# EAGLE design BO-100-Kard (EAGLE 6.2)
PLPB#: PLPB-0046; REV: X1
Assembly variants: build

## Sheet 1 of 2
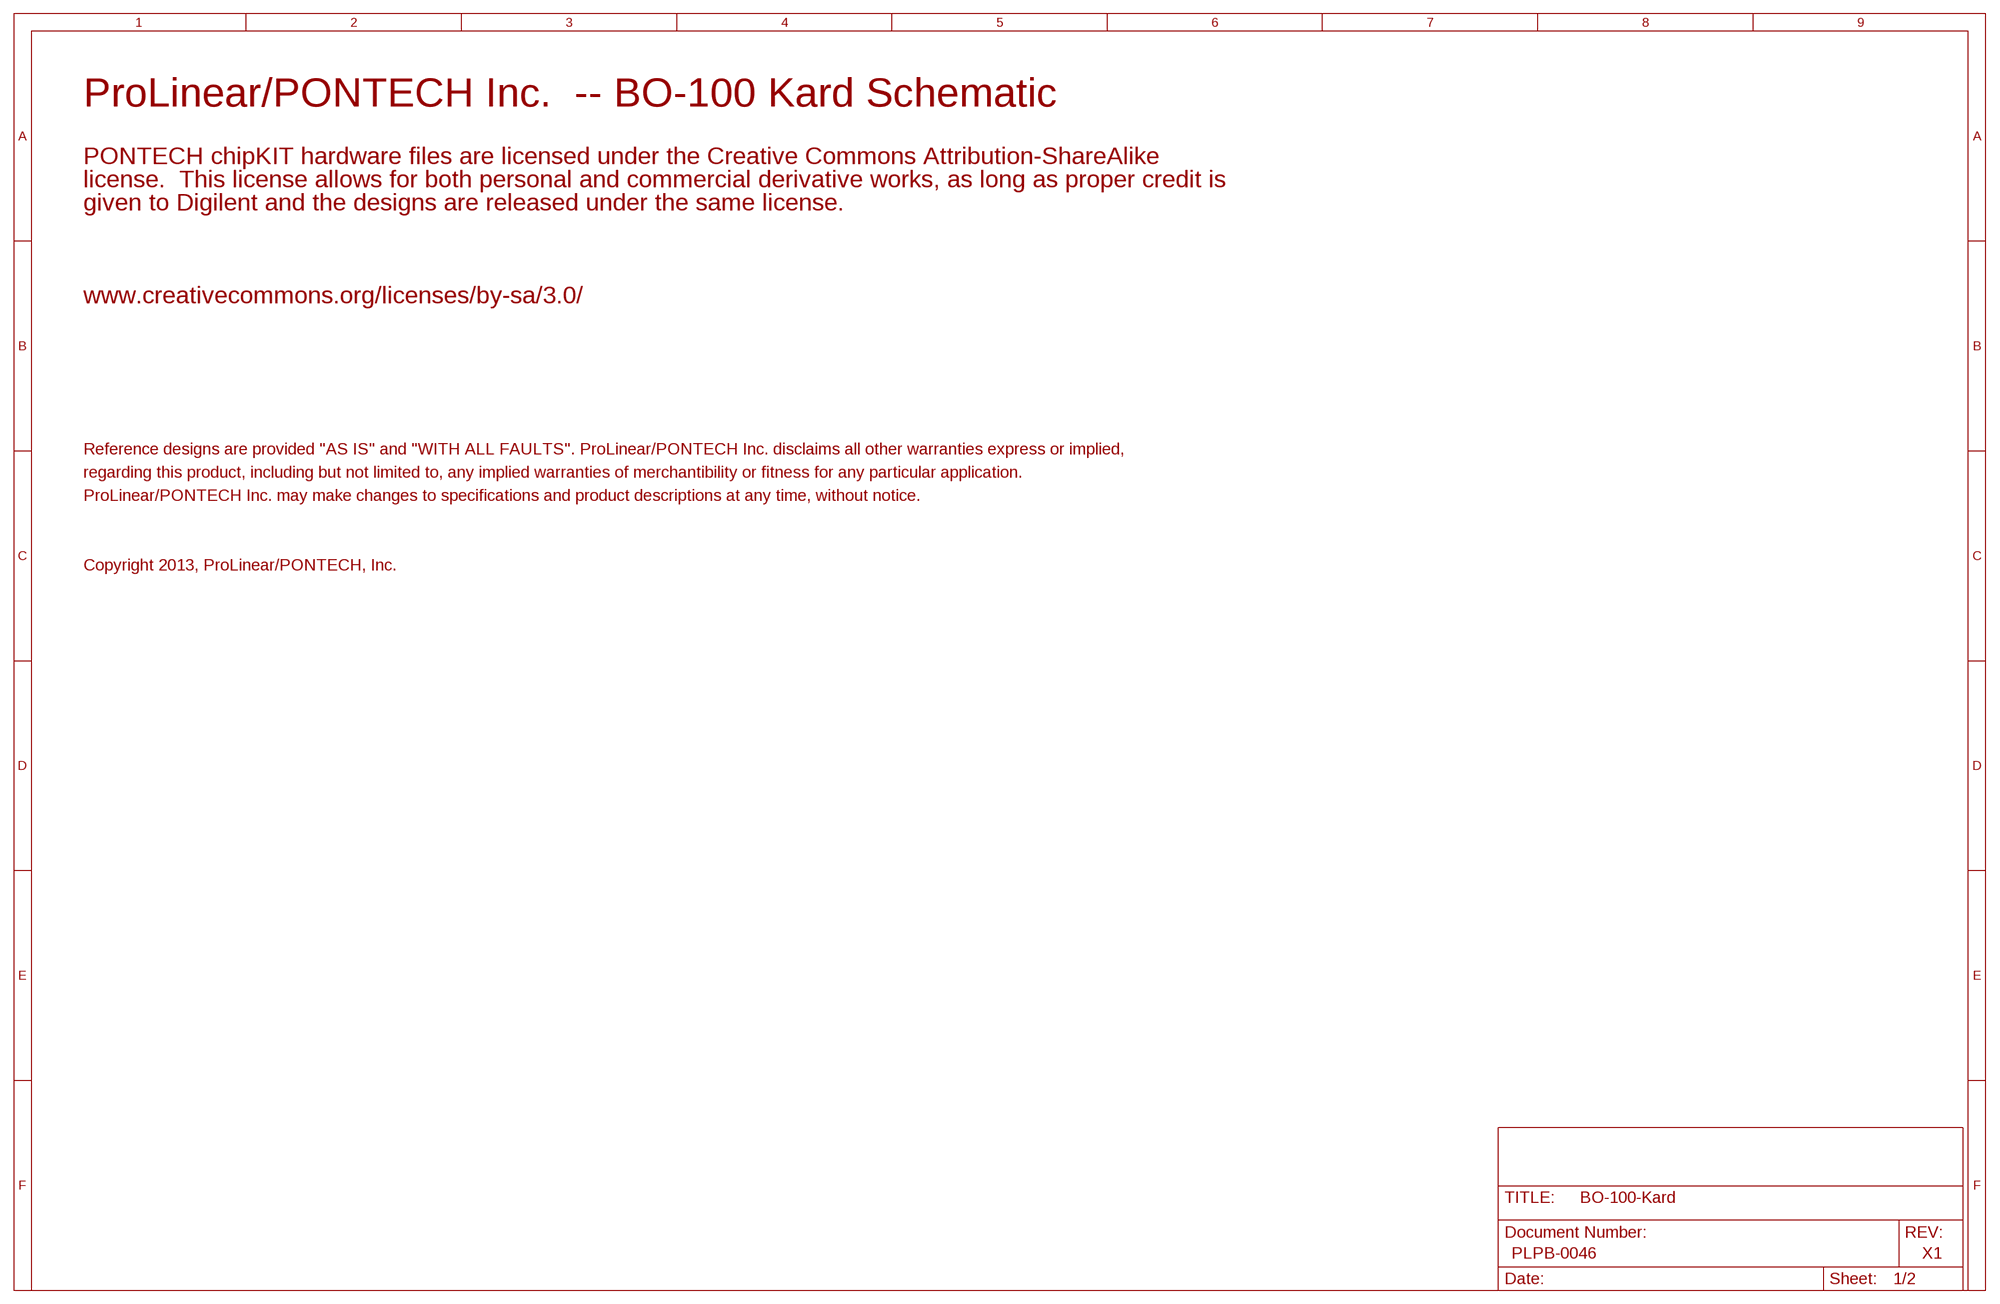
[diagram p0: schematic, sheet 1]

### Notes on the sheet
- ProLinear/PONTECH Inc.  -- BO-100 Kard Schematic
- PONTECH chipKIT hardware files are licensed under the Creative Commons Attribution-ShareAlike
- license.  This license allows for both personal and commercial derivative works, as long as proper credit is
- given to Digilent and the designs are released under the same license.
- www.creativecommons.org/licenses/by-sa/3.0/
- Reference designs are provided "AS IS" and "WITH ALL FAULTS". ProLinear/PONTECH Inc. disclaims all other warranties express or implied,
- regarding this product, including but not limited to, any implied warranties of merchantibility or fitness for any particular application.
- ProLinear/PONTECH Inc. may make changes to specifications and product descriptions at any time, without notice.
- Copyright 2013, ProLinear/PONTECH, Inc.

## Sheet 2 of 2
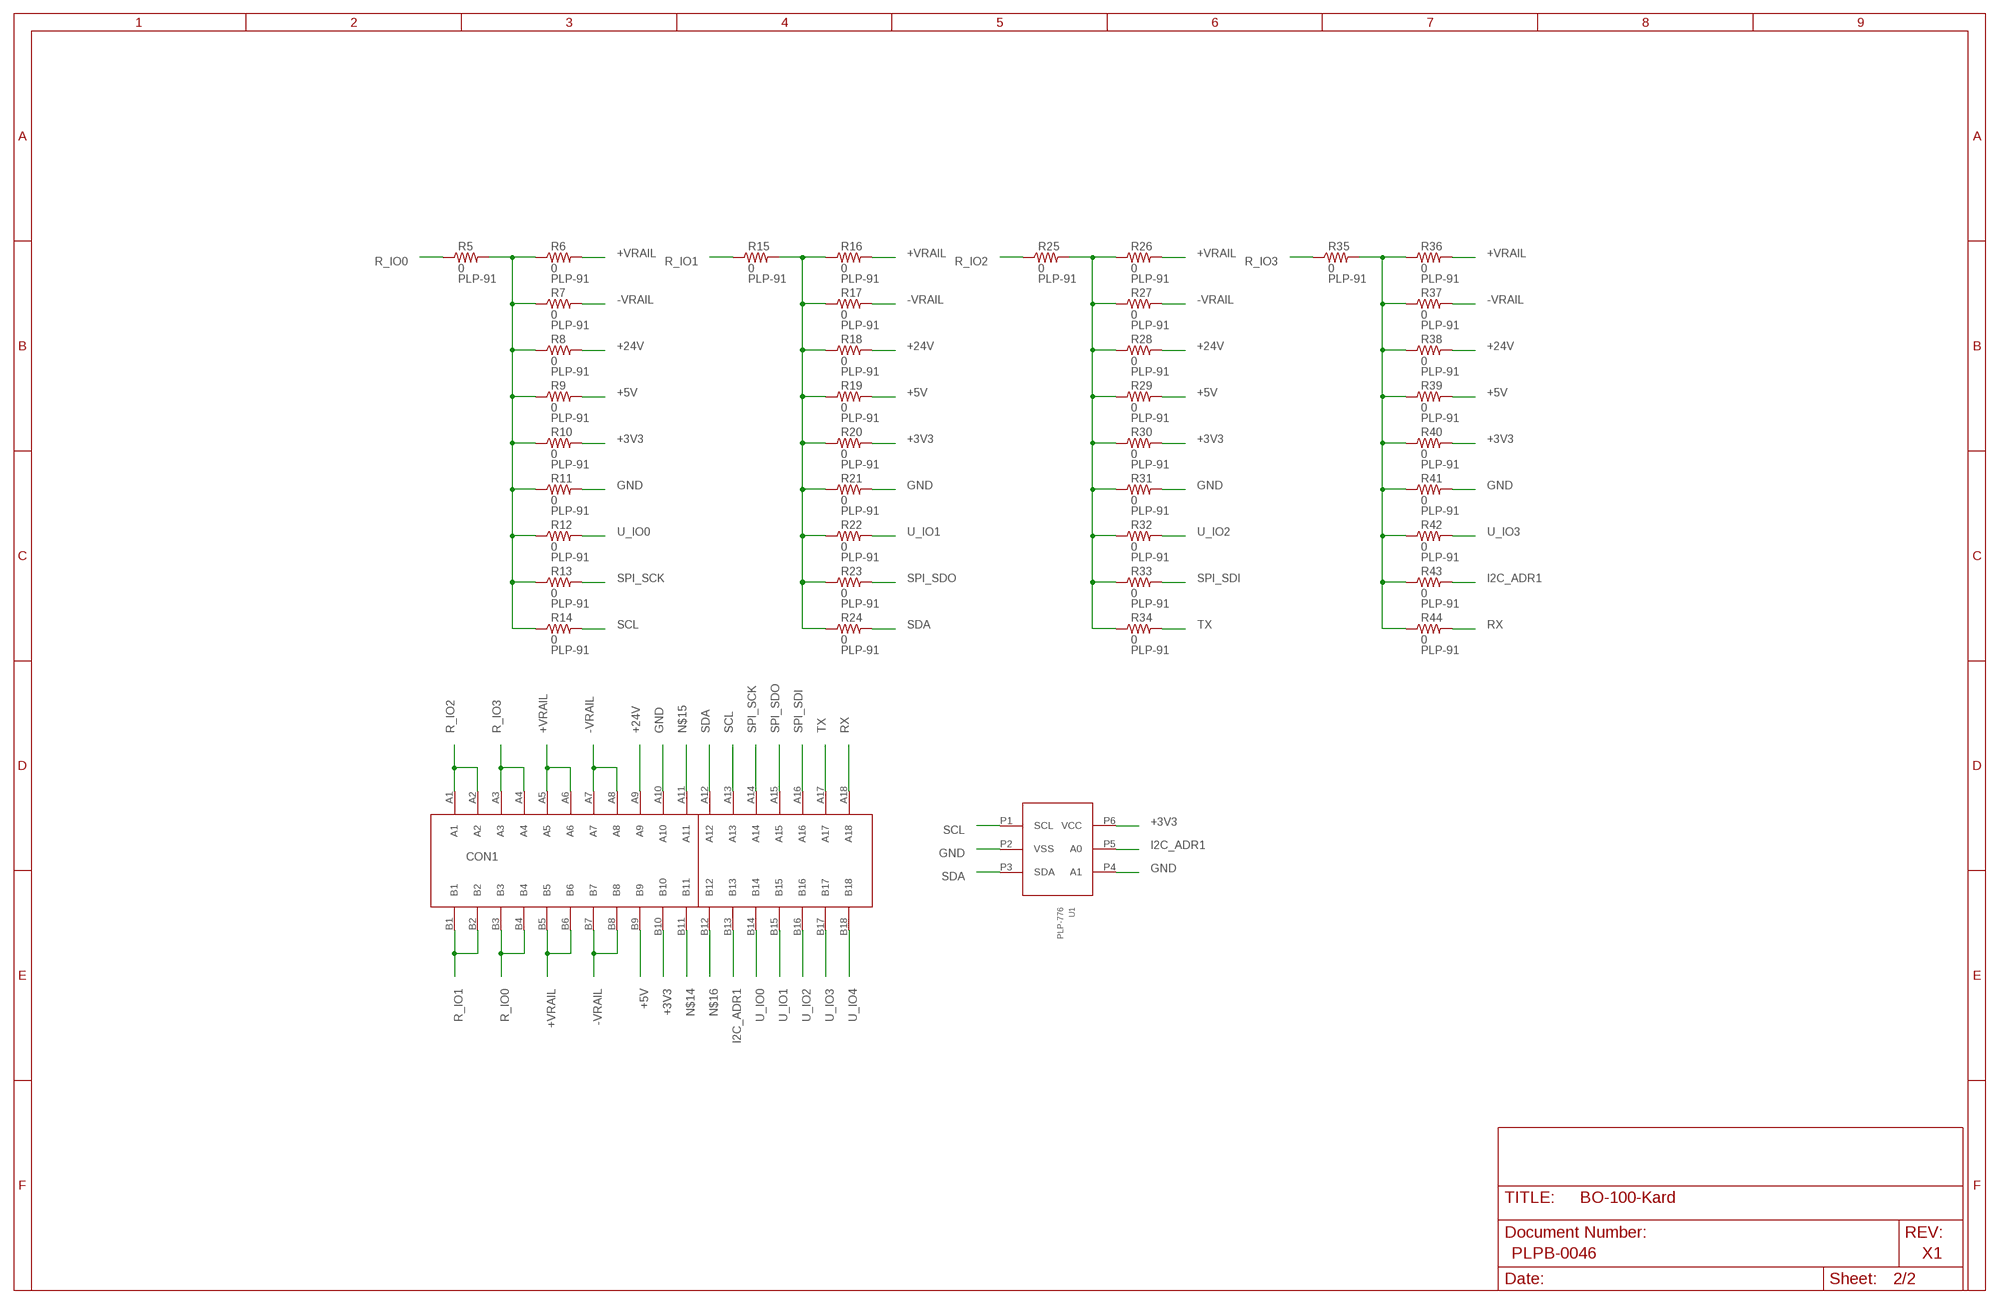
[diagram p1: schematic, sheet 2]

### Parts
CON1  PLPA-0107  [PLPA-0107]
R5  0  PLP-91  [DISCRETE_R0603]
R6  0  PLP-91  [DISCRETE_R0603]
R7  0  PLP-91  [DISCRETE_R0603]
R8  0  PLP-91  [DISCRETE_R0603]
R9  0  PLP-91  [DISCRETE_R0603]
R10  0  PLP-91  [DISCRETE_R0603]
R11  0  PLP-91  [DISCRETE_R0603]
R12  0  PLP-91  [DISCRETE_R0603]
R13  0  PLP-91  [DISCRETE_R0603]
R14  0  PLP-91  [DISCRETE_R0603]
R15  0  PLP-91  [DISCRETE_R0603]
R16  0  PLP-91  [DISCRETE_R0603]
R17  0  PLP-91  [DISCRETE_R0603]
R18  0  PLP-91  [DISCRETE_R0603]
R19  0  PLP-91  [DISCRETE_R0603]
R20  0  PLP-91  [DISCRETE_R0603]
R21  0  PLP-91  [DISCRETE_R0603]
R22  0  PLP-91  [DISCRETE_R0603]
R23  0  PLP-91  [DISCRETE_R0603]
R24  0  PLP-91  [DISCRETE_R0603]
R25  0  PLP-91  [DISCRETE_R0603]
R26  0  PLP-91  [DISCRETE_R0603]
R27  0  PLP-91  [DISCRETE_R0603]
R28  0  PLP-91  [DISCRETE_R0603]
R29  0  PLP-91  [DISCRETE_R0603]
R30  0  PLP-91  [DISCRETE_R0603]
R31  0  PLP-91  [DISCRETE_R0603]
R32  0  PLP-91  [DISCRETE_R0603]
R33  0  PLP-91  [DISCRETE_R0603]
R34  0  PLP-91  [DISCRETE_R0603]
R35  0  PLP-91  [DISCRETE_R0603]
R36  0  PLP-91  [DISCRETE_R0603]
R37  0  PLP-91  [DISCRETE_R0603]
R38  0  PLP-91  [DISCRETE_R0603]
R39  0  PLP-91  [DISCRETE_R0603]
R40  0  PLP-91  [DISCRETE_R0603]
R41  0  PLP-91  [DISCRETE_R0603]
R42  0  PLP-91  [DISCRETE_R0603]
R43  0  PLP-91  [DISCRETE_R0603]
R44  0  PLP-91  [DISCRETE_R0603]
U1  PLP-776  [SOT23-6]

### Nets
+3V3 [Power]: CON1.B10 R10.2 R20.2 R30.2 R40.2 U1.P6(VCC)
+5V [Power]: CON1.B9 R9.2 R19.2 R29.2 R39.2
+24V [Power]: CON1.A9 R8.2 R18.2 R28.2 R38.2
+VRAIL [Power]: CON1.A5 CON1.A6 CON1.B5 CON1.B6 R6.2 R16.2 R26.2 R36.2
-VRAIL [Power]: CON1.A7 CON1.A8 CON1.B7 CON1.B8 R7.2 R17.2 R27.2 R37.2
GND [Power]: CON1.A10 R11.2 R21.2 R31.2 R41.2 U1.P2(VSS) U1.P4(A1)
I2C_ADR1: CON1.B13 R43.2 U1.P5(A0)
N$5 [Power]: R5.2 R6.1 R7.1 R8.1 R9.1 R10.1 R11.1 R12.1 R13.1 R14.1
N$6 [Power]: R15.2 R16.1 R17.1 R18.1 R19.1 R20.1 R21.1 R22.1 R23.1 R24.1
N$7 [Power]: R25.2 R26.1 R27.1 R28.1 R29.1 R30.1 R31.1 R32.1 R33.1 R34.1
N$8 [Power]: R35.2 R36.1 R37.1 R38.1 R39.1 R40.1 R41.1 R42.1 R43.1 R44.1
N$14: CON1.B11
N$15: CON1.A11
N$16: CON1.B12
R_IO0 [Power]: CON1.B3 CON1.B4 R5.1
R_IO1 [Power]: CON1.B1 CON1.B2 R15.1
R_IO2 [Power]: CON1.A1 CON1.A2 R25.1
R_IO3 [Power]: CON1.A3 CON1.A4 R35.1
RX: CON1.A18 R44.2
SCL: CON1.A13 R14.2 U1.P1(SCL)
SDA: CON1.A12 R24.2 U1.P3(SDA)
SPI_SCK: CON1.A14 R13.2
SPI_SDI: CON1.A16 R33.2
SPI_SDO: CON1.A15 R23.2
TX: CON1.A17 R34.2
U_IO0: CON1.B14 R12.2
U_IO1: CON1.B15 R22.2
U_IO2: CON1.B16 R32.2
U_IO3: CON1.B17 R42.2
U_IO4: CON1.B18

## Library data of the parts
CON1 = PLP:PLPA-0107: CONN PCI EXPRESS 36POS VERT PCB; PLP#: PLPA-0107
R5-R44 = PLP:PLP-91: Resistor; PLP#: PLP-91
U1 = PLP:PLP-776: IC EEPROM 2KBIT 400KHZ SOT23-6; PLP#: PLP-776

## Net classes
1 Power: width 0.254 mm

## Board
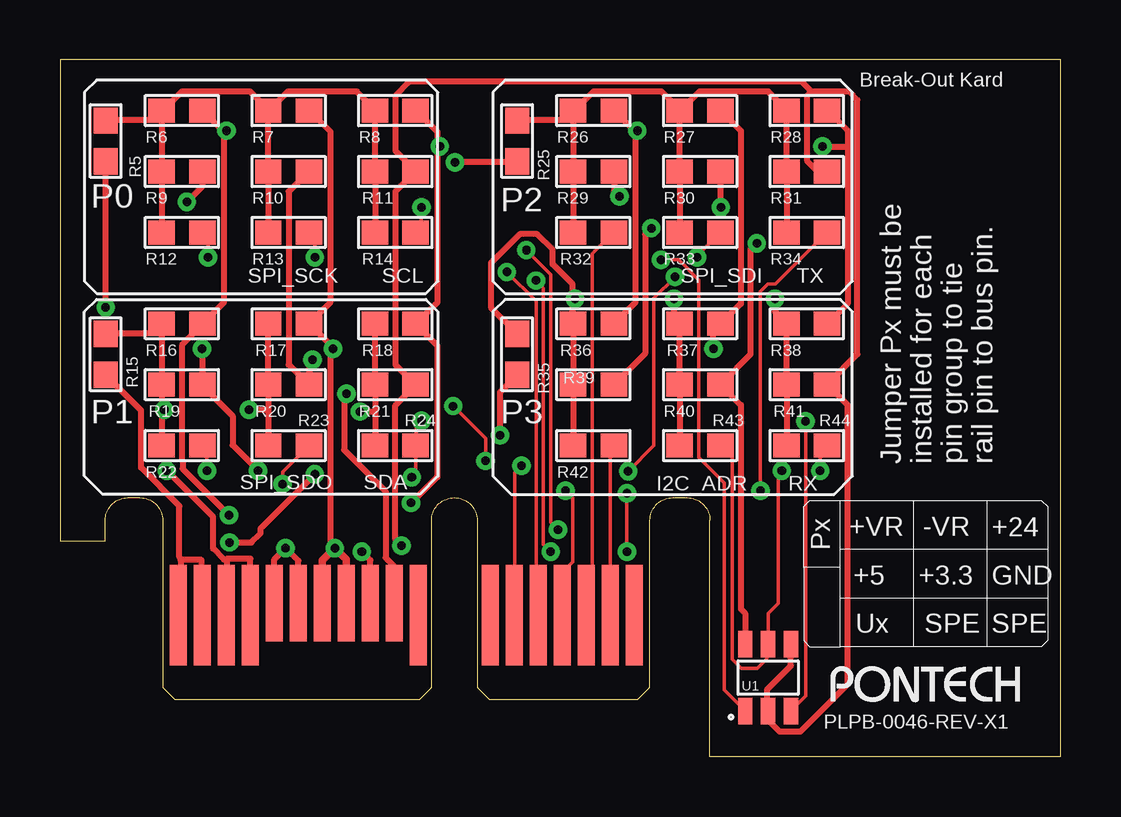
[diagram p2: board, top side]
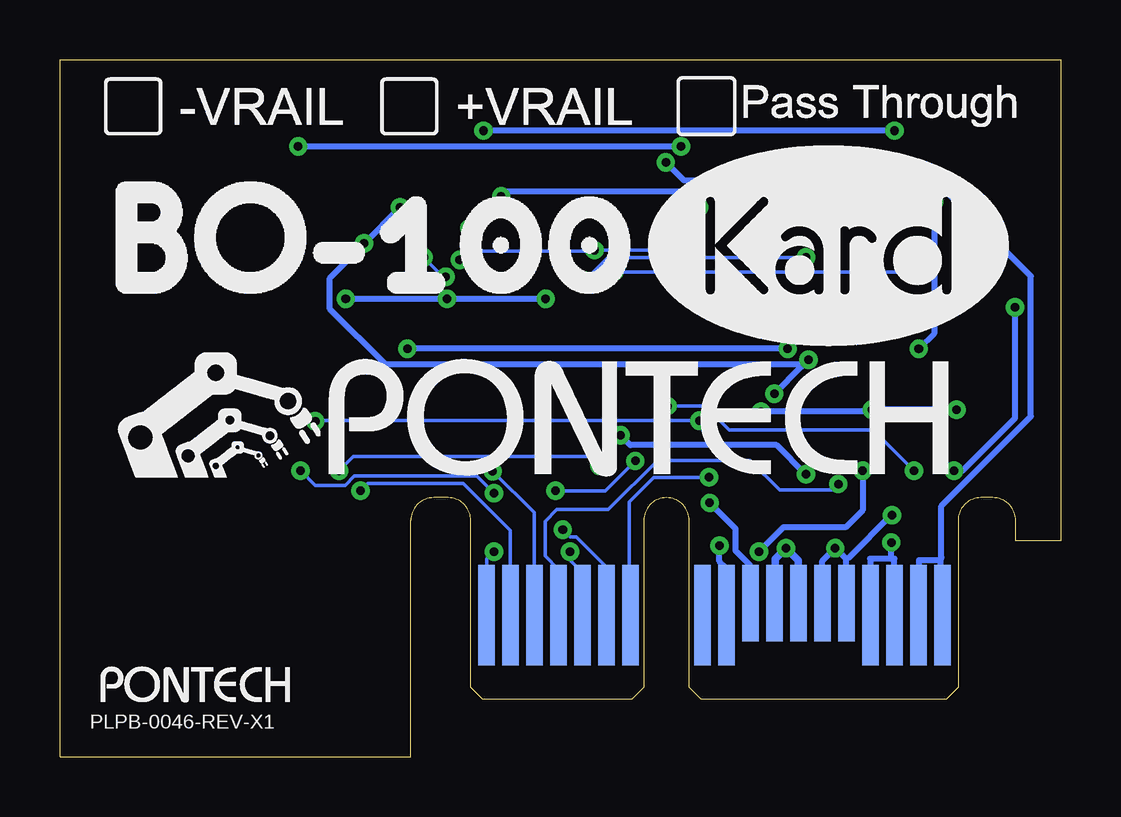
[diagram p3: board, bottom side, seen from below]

Size 41.7 x 29.05 mm. Coordinates in mm from the lower left corner, seen from the top.
Outline: 1.88,9.85 1.88,9 0,9 0,29.05 41.7,29.05 41.7,0 27.08,0 27.08,9.85
Copper layers (1*16): Top 0.0178mm / dielectric 59mil / Bottom 0.0178mm
Design rules: minimum track width 6mil, minimum drill 14mil, track to track 6mil, track to pad 6mil, pad to pad 6mil, via to via 6mil, smd to smd 6mil, copper to edge 20mil, drill to drill 16mil, minimum pad ring 8mil, minimum via ring 8mil, stop-mask expansion 3mil, vias tented up to drill 14mil, thermal gap 10mil
tKeepout: area 0,-1 to 0.8,29.1; area 41,-1 to 41.7,29.1
bKeepout: area 0,-1 to 0.8,29.1; area 41,-1 to 41.7,29.1

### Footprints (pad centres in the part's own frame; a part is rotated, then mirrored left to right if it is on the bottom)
PLPA-0107 = smd 0.7 x 4.2 bottom: A1 -11.5,3.5; A2 -10.5,3.5; A3 -9.5,3.5; A4 -8.5,3.5; A10 -2.5,3.5; A11 -1.5,3.5; A12 1.5,3.5; A13 2.5,3.5; A14 3.5,3.5; A15 4.5,3.5; A16 5.5,3.5; A17 6.5,3.5; A18 7.5,3.5 | smd 0.7 x 3.2 bottom: A5 -7.5,4; A6 -6.5,4; A7 -5.5,4; A8 -4.5,4; A9 -3.5,4 | smd 0.7 x 4.2: B1 -11.5,3.5; B2 -10.5,3.5; B3 -9.5,3.5; B4 -8.5,3.5; B11 -1.5,3.5; B12 1.5,3.5; B13 2.5,3.5; B14 3.5,3.5; B15 4.5,3.5; B16 5.5,3.5; B17 6.5,3.5; B18 7.5,3.5 | smd 0.7 x 3.2: B5 -7.5,4; B6 -6.5,4; B7 -5.5,4; B8 -4.5,4; B9 -3.5,4; B10 -2.5,4
DISCRETE_R0603 = smd 1.1 x 1: 1 -0.85,0; 2 0.85,0
SOT23-6 = smd 0.6 x 1.1: P1 -0.95,-1.4; P2 0,-1.4; P3 0.95,-1.4; P4 0.95,1.4; P5 0,1.4; P6 -0.95,1.4

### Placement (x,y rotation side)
CON1  16.43,2.4 0 top
R5  1.91,25.67 90 top
R6  5.08,26.94 0 top
R7  9.53,26.94 0 top
R8  13.97,26.94 0 top
R9  5.08,24.4 0 top
R10  9.53,24.4 0 top
R11  13.97,24.4 0 top
R12  5.08,21.86 0 top
R13  9.53,21.86 0 top
R14  13.97,21.86 0 top
R15  1.91,16.78 90 top
R16  5.08,18.05 0 top
R17  9.53,18.05 0 top
R18  13.97,18.05 0 top
R19  5.08,15.51 0 top
R20  9.53,15.51 0 top
R21  13.97,15.51 0 top
R22  5.08,12.97 0 top
R23  9.53,12.97 0 top
R24  13.97,12.97 0 top
R25  19.05,25.67 90 top
R26  22.23,26.94 0 top
R27  26.67,26.94 0 top
R28  31.11,26.94 0 top
R29  22.23,24.4 0 top
R30  26.67,24.4 0 top
R31  31.11,24.4 0 top
R32  22.23,21.86 0 top
R33  26.67,21.86 0 top
R34  31.11,21.86 0 top
R35  19.05,16.78 90 top
R36  22.23,18.05 0 top
R37  26.67,18.05 0 top
R38  31.11,18.05 0 top
R39  22.23,15.51 0 top
R40  26.67,15.51 0 top
R41  31.11,15.51 0 top
R42  22.23,12.97 0 top
R43  26.67,12.97 0 top
R44  31.11,12.97 0 top
U1  29.5,3.3 0 top
U$1  [PONTECH-LOGO-LARGE]  4.57,11.7 0 bottom
U$2  [PONTECH-TEXT]  40,2.3 0 top
U$3  [PONTECH-TEXT]  32.12,2.29 0 bottom
U$5  [BO-100]  39.37,19.32 0 bottom
U$7  [PASSTHROUGH_VRAIL_CHECK]  39.92,25.92 0 bottom

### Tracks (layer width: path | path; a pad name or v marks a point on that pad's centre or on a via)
+3V3  (via drill 0.36)
  Top 0.254: 28.55,4.71 U1.P6 28.55,5.99 28.37,6.16 28.37,14.67 27.53,15.51 R40.2 27.61,15.61 28.78,16.78 28.78,21.15 v29.03,21.4 | v27.53,22.9 27.53,24.4 R30.2 | R10.2 10.36,24.4 9.53,23.56 9.53,16.35 10.36,15.51 R20.2 10.38,16.41 v10.52,16.55 | v11.94,15.13 11.84,15.03 11.84,12.79 13.56,11.06 13.56,8.3 13.92,7.94 13.92,6.42 CON1.B10
  Bottom 0.254: v27.53,22.9 v29.03,21.4 29.11,21.3 30.45,19.95 30.45,18.67 28.14,16.35 10.9,16.35 10.81,16.26 | v10.52,16.55 10.81,16.26 | 10.81,16.26 v11.94,15.13
+5V  (via drill 0.36)
  Top 0.254: v24.64,22.04 24.38,21.78 24.38,16.8 R39.2 | v23.32,23.36 23.09,23.59 R29.2 | v5.92,17.01 5.92,15.51 R19.2 5.99,15.41 7.19,14.21 7.19,12.99 v8.26,11.93 | v5.28,23.13 5.92,23.77 5.92,24.4 R9.2 | v12.57,8.55 12.93,8.2 12.93,6.42 CON1.B9
  Bottom 0.254: v24.64,22.04 v23.32,23.36 23.22,23.43 23.09,23.56 5.74,23.56 5.38,23.21 v5.28,23.13 5.28,17.64 v5.92,17.01 | v8.26,11.93 8.26,10.28 8.97,9.57 11.56,9.57 v12.57,8.55
+24V  (via drill 0.36)
  Top 0.254: 32.82,25.44 32.82,26.1 31.98,26.94 R28.2 | 32.82,25.44 32.82,18.89 31.98,18.05 R38.2 | 15.72,25.44 15.72,26.05 14.83,26.94 R8.2 | 15.72,25.44 15.72,18.94 14.83,18.05 R18.2 14.91,17.95 15.72,17.14 15.72,11.65 15.7,11.65 v14.63,10.58 | v31.77,25.44 32.82,25.44 | v15.82,25.44 15.72,25.44
  Bottom 0.254: v14.63,10.58 13.56,9.52 13.56,8.6 12.95,7.99 12.95,6.42 CON1.A9 | v15.82,25.44 v31.77,25.44
+VRAIL  (via drill 0.36)
  Top 0.254: CON1.A6 9.93,8.17 v9.4,8.7 8.93,8.23 CON1.A5 | 23.98,26.05 23.98,18.94 R36.2 | 23.98,26.05 R26.2 | 6.83,26.05 6.83,18.94 5.94,18.05 R16.2 5.87,17.95 5.08,17.16 5.08,12.36 5.11,12.34 5.11,12.01 v7.04,10.07 | 6.83,26.05 5.94,26.94 R6.2 | v24.05,26.1 23.98,26.05 | v6.93,26.1 6.83,26.05
  Bottom 0.254: 8.95,8.25 v9.4,8.7 9.93,8.17 CON1.A6 | CON1.A5 8.95,5.92 8.95,8.25 | v7.04,10.07 7.06,10.07 8.84,8.3 8.95,8.25 | v6.93,26.1 v24.05,26.1
-VRAIL  (via drill 0.36)
  Top 0.254: R27.2 27.53,26.94 28.37,26.1 28.37,18.89 27.53,18.05 R37.2 27.46,17.95 27.23,17.72 v27.23,17.01 | 11.28,17.01 11.28,8.73 v11.45,8.7 | 11.28,17.01 11.28,17.16 R17.2 10.46,18.15 11.28,18.96 11.28,26.05 R7.2 | v11.38,17.01 11.28,17.01
  Top 0.305: CON1.A7 10.93,8.18 v11.45,8.7 11.93,8.22 CON1.A8
  Bottom 0.254: v11.38,17.01 v27.23,17.01
  Bottom 0.305: CON1.A8 11.93,6.82 11.9,6.85 11.9,8.25 v11.45,8.7 10.93,8.18 CON1.A7
GND  (via drill 0.36)
  Top 0.254: 30.43,4.36 30.43,4.69 U1.P4 30.45,3.8 29.46,2.81 29.46,1.94 U1.P2 | 29.52,1.92 U1.P2 | R31.2 31.57,24.4 31.11,24.86 31.11,27.55 31.29,27.73 | 31.29,27.73 32.88,27.73 33.22,27.38 33.22,16.78 32.05,15.61 R41.2 31.98,15.51 32.82,14.67 32.82,3.01 30.86,1.06 29.97,1.06 29.57,1.46 29.57,1.79 29.5,1.86 U1.P2 | 31.29,27.73 31.22,27.83 30.91,28.13 14.55,28.13 13.97,27.55 13.97,25.26 14.73,24.5 R11.2 14.81,24.4 13.97,23.56 13.97,16.35 14.81,15.51 R21.2 14.73,15.41 13.97,14.65 13.97,9.06 v14.22,8.8
  Bottom 0.254: CON1.A10 13.95,5.91 13.95,7.87 14.22,8.14 v14.22,8.8
I2C_ADR1  (via drill 0.36)
  Top 0.152: v30.07,11.93 29.92,11.78 29.92,6.39 29.5,5.97 U1.P5 29.44,4.66 29.44,4.08 29.05,3.69 28.38,3.69 28.02,4.05 28.02,12.49 27.53,12.97 R43.2 | v19.23,12.13 18.95,11.85 18.95,5.91 CON1.B13
  Bottom 0.152: v30.07,11.93 29.49,12.51 19.61,12.51 v19.23,12.13
N$5
  Top 0.254: R12.1 4.24,21.86 4.24,24.4 R9.1 4.24,24.5 4.24,26.43 4.22,26.53 | 4.22,26.53 1.91,26.53 R5.2 | 4.22,26.53 4.22,26.94 R6.1 4.34,26.99 5.08,27.73 7.92,27.73 8.61,27.04 R7.1 | R13.1 R10.1 8.69,24.5 R7.1 | R14.1 13.13,21.86 13.13,24.4 R11.1 13.13,24.5 13.13,26.94 R8.1 13.06,27.04 12.37,27.73 9.5,27.73 8.79,27.02 R7.1
N$6  (via drill 0.36)
  Top 0.254: 13.13,14.39 13.13,15.51 R21.1 13.13,15.61 13.13,18.05 R18.1 | 13.13,14.39 13.13,12.97 R24.1 | 8.69,14.47 R20.1 8.69,15.61 R17.1 | 8.69,14.47 R23.1 | 4.24,14.47 4.24,15.51 R19.1 4.24,15.61 4.24,17.54 4.22,17.64 | 4.24,14.47 4.24,12.97 R22.1 | 4.22,17.64 1.91,17.64 R15.2 | 4.22,17.64 4.22,18.05 R16.1 | v7.87,14.47 8.69,14.47 | v4.34,14.47 4.24,14.47 | v12.5,14.39 13.13,14.39
  Bottom 0.254: v4.34,14.47 v7.87,14.47 7.98,14.39 v12.5,14.39
N$7
  Top 0.254: R32.1 R29.1 21.39,24.5 21.39,26.43 21.36,26.53 | 21.36,26.53 19.05,26.53 R25.2 | 21.36,26.53 21.36,26.94 R26.1 21.49,26.99 22.23,27.73 25.07,27.73 25.76,27.04 R27.1 | R33.1 25.83,21.86 25.83,24.4 R30.1 25.83,24.5 25.83,26.94 R27.1 | R34.1 30.28,21.86 30.28,24.4 R31.1 30.28,24.5 30.28,26.94 R28.1 30.2,27.04 29.52,27.73 26.64,27.73 25.93,27.02 R27.1
N$8  (via drill 0.36)
  Top 0.254: R44.1 30.28,12.97 30.28,15.51 R41.1 30.28,15.61 30.28,18.05 R38.1 30.2,18.15 29.79,18.56 v29.79,19.09 | R43.1 25.83,12.97 25.83,15.51 R40.1 25.83,15.61 25.83,18.05 R37.1 25.76,18.15 25.58,18.33 v25.58,19.09 | R42.1 R39.1 21.39,15.61 21.39,17.95 R36.1 21.36,18.05 21.36,19.09 | 21.36,19.09 21.36,19.7 20.52,20.54 20.52,21.16 19.89,21.78 19.15,21.78 17.96,20.59 17.96,18.74 19.05,17.64 R35.2 | v21.46,19.09 21.36,19.09
  Bottom 0.254: v21.46,19.09 v25.58,19.09 v29.79,19.09
R_IO0  (via drill 0.36)
  Top 0.254: CON1.B4 7.93,8.25 6.95,8.25 6.95,8.22 | 6.95,8.22 6.95,5.9 CON1.B3 | v4.45,11.93 6.38,10 6.38,8.68 6.83,8.22 6.95,8.22 | v1.91,18.74 R5.1
  Bottom 0.254: v1.91,18.74 1.91,14.11 4.09,11.93 v4.45,11.93
R_IO1
  Top 0.254: CON1.B2 5.9,8.2 5.03,8.2 | 5.03,8.2 5.03,5.9 CON1.B1 5.05,5.9 | R15.1 1.91,15.92 3.38,14.44 3.38,12.06 4.98,10.46 4.98,8.32 5.03,8.2
R_IO2  (via drill 0.36)
  Top 0.254: v16.46,24.78 16.46,24.81 19.05,24.81 R25.1
  Bottom 0.254: CON1.A2 5.9,5.9 5.9,8.2 5.03,8.2 | 5.03,8.2 5.03,6.4 CON1.A1 | v16.46,24.78 15.7,24.02 5.23,24.02 1.25,20.03 1.25,14.19 4.98,10.46 4.98,8.32 5.03,8.2
R_IO3  (via drill 0.36)
  Top 0.254: v18.34,13.4 18.34,15.2 19.05,15.92 R35.1 | v10.62,11.78 8.36,9.52 8.36,9.31 7.98,8.93 v7.06,8.93
  Bottom 0.254: CON1.A3 6.93,8.25 7.06,8.25 | 7.06,8.25 7.95,8.25 7.95,5.95 CON1.A4 | v18.34,13.4 17.93,12.99 11.84,12.99 v10.62,11.78 | 7.06,8.25 v7.06,8.93
RX  (via drill 0.36)
  Top 0.152: v31.67,11.93 31.67,12.69 R44.2 | v23.62,8.55 v23.62,10.99
  Bottom 0.152: v31.67,11.93 31.06,11.32 29.82,11.32 29.44,11.7 24.33,11.7 v23.62,10.99 | CON1.A18 23.93,8.25 v23.62,8.55
SCL  (via drill 0.36)
  Top 0.152: v15.06,22.9 15.06,22.09 14.83,21.86 R14.2 | v19.43,21.12 20.45,20.11 20.45,9.77 v20.75,9.46 | v25.04,20.72 25.78,20.72 26.62,19.88 26.62,12.49 27.69,11.42 27.69,2.79 28.55,1.92 U1.P1
  Bottom 0.152: v15.06,22.9 16.84,21.12 v19.43,21.12 19.48,21.07 24.69,21.07 v25.04,20.72 | v20.75,9.46 20.45,9.16 20.19,9.16 18.95,7.91 18.95,5.91 CON1.A13
SDA  (via drill 0.36)
  Top 0.152: v31.06,13.99 31.06,2.53 30.45,1.92 U1.P3 | v15.06,14.01 14.83,13.78 14.83,12.97 R24.2 | 14.88,12.92 R24.2 | v14.66,11.65 14.82,11.81 R24.2
  Bottom 0.152: v31.06,13.99 31.04,14.01 v15.06,14.01 | CON1.A12 17.98,5.96 17.98,10.62 16.95,11.65 v14.66,11.65
  Bottom 0.155: 18,5.9 CON1.A12
SPI_SCK  (via drill 0.36)
  Top 0.152: v10.62,20.82 10.62,21.63 R13.2 | v19.84,19.85 20.14,19.55 20.14,8.86 v20.45,8.55
  Bottom 0.152: v10.62,20.82 18.87,20.82 v19.84,19.85 | v20.45,8.55 20.45,8.2 19.94,7.69 CON1.A14
SPI_SDI  (via drill 0.36)
  Top 0.152: v26.54,20.82 26.54,20.89 27.51,21.86 R33.2 | v25.63,20.01 24.74,19.12 24.74,12.97 v23.67,11.9
  Bottom 0.152: v26.54,20.82 25.73,20.01 v25.63,20.01 | v23.67,11.9 21.95,10.18 21.95,5.91 CON1.A16
SPI_SDO  (via drill 0.36)
  Top 0.152: v9.27,11.37 9.27,11.87 R23.2
  Bottom 0.152: CON1.A15 20.93,7.81 21.49,8.37 21.49,9.82 21.01,10.3 18.85,10.3 16.79,12.36 12.95,12.36 11.71,11.12 9.53,11.12 v9.27,11.37
TX  (via drill 0.36)
  Top 0.152: v29.18,11.09 29.18,19.39 29.49,19.7 29.79,19.7 R34.2
  Bottom 0.152: v29.18,11.09 28.88,11.39 24.89,11.39 22.94,9.44 CON1.A17
U_IO0  (via drill 0.36)
  Top 0.152: v6.17,20.82 6.17,21.63 5.94,21.86 R12.2 | v18.62,20.21 19.84,18.99 19.84,5.99 19.91,5.91 CON1.B14
  Bottom 0.152: v6.17,20.82 6.78,20.21 v18.62,20.21
U_IO1  (via drill 0.36)
  Top 0.152: v6.12,11.93 6.12,12.79 5.94,12.97 R22.2 | v16.38,14.62 17.73,13.28 v17.73,12.34 | v21.06,11.09 21.36,10.79 21.36,8.12 20.95,7.71 20.95,5.91 CON1.B15
  Bottom 0.152: v6.12,11.93 7.82,13.63 13.82,13.63 14.81,14.62 v16.38,14.62 | v21.06,11.09 18.97,11.09 v17.73,12.34
U_IO2
  Top 0.152: R32.2 23.06,21.86 22.17,20.97 22.17,6.14 21.95,5.91 CON1.B16
U_IO3
  Top 0.152: R42.2 23.06,12.97 22.94,12.84 22.94,6.47 CON1.B17
  Top 0.155: 22.95,6.35 22.9,6.4 CON1.B17

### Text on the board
tPlace: Break-Out Kard | P0 | P2 | SPI_SCK | SCL | SPI_SDI | TX | P1 | P3 | Jumper Px must be | installed for each | pin group to tie | rail pin to bus pin. | SPI_SDO | SDA | I2C_ADR | RX | Px | +VR | -VR | +24 | +5 | +3.3 | GND | Ux | SPE | SPE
